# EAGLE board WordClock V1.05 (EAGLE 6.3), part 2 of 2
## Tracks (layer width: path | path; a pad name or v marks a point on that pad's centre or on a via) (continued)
LED13@U1  (via drill 0.5) (continued)
  Bottom 0.254: U101.27 145.25,352.19 145.77,351.66 v145.77,350.65
LED13@U2  (via drill 0.5)
  Top 0.406: v145.77,288.65 146.03,288.39 234.29,288.39 238.86,283.82 238.86,283.33 D220.C
  Bottom 0.254: U201.27 145.25,290.19 145.77,289.66 v145.77,288.65
LED13@U3  (via drill 0.5)
  Top 0.406: v145.77,226.65 146.03,226.39 234.29,226.39 238.86,221.82 238.86,221.33 D320.C
  Bottom 0.254: U301.27 145.25,228.19 145.77,227.66 v145.77,226.65
LED13@U4  (via drill 0.5)
  Top 0.406: v145.77,164.65 146.03,164.39 234.29,164.39 238.86,159.82 238.86,159.33 D420.C
  Bottom 0.254: U401.27 145.25,166.19 145.77,165.66 v145.77,164.65
LED13@U5  (via drill 0.5)
  Top 0.406: v145.77,102.65 146.03,102.39 154.44,102.39 156.44,104.39 156.44,110.49 158.34,112.39 237.59,112.39 239.3,110.69 D520.C
  Bottom 0.254: U501.27 145.25,104.19 145.77,103.66 v145.77,102.65
LED14@U1  (via drill 0.5)
  Top 0.406: v145.01,351.41 145.01,350.14 145.52,349.63 207.11,349.63 211.18,345.57 211.18,344.91 D119.C
  Bottom 0.254: U101.28 144.75,351.67 v145.01,351.41
LED14@U2  (via drill 0.5)
  Top 0.406: v145.01,289.41 145.01,288.14 145.52,287.63 207.11,287.63 211.18,283.57 211.18,282.91 D219.C
  Bottom 0.254: U201.28 144.75,289.67 v145.01,289.41
LED14@U3  (via drill 0.5)
  Top 0.406: v145.01,227.41 145.01,226.14 145.52,225.63 207.11,225.63 211.18,221.57 211.18,220.91 D319.C
  Bottom 0.254: U301.28 144.75,227.67 v145.01,227.41
LED14@U4  (via drill 0.5)
  Top 0.406: v145.01,165.41 145.01,164.14 145.52,163.63 207.11,163.63 211.18,159.57 211.18,158.91 D419.C
  Bottom 0.254: U401.28 144.75,165.67 v145.01,165.41
LED14@U5  (via drill 0.5)
  Top 0.406: v145.01,103.41 145.01,102.14 145.52,101.63 207.11,101.63 211.18,97.57 211.18,96.91 D519.C
  Bottom 0.254: U501.28 144.75,103.67 v145.01,103.41
LED15@U1  (via drill 0.5)
  Top 0.406: D118.C 182.86,345.13 182.86,345.69 179.81,348.74 145.26,348.74 144.25,349.76 v144.25,350.64 v144.25,350.65
  Bottom 0.254: U101.29 v144.25,350.65
LED15@U2  (via drill 0.5)
  Top 0.406: D218.C 182.86,283.13 182.86,283.69 179.81,286.74 145.26,286.74 144.25,287.76 144.25,288.01 144.25,288.02 v144.25,288.65
  Bottom 0.254: U201.29 v144.25,288.65
LED15@U3  (via drill 0.5)
  Top 0.406: D318.C 182.86,221.13 182.86,221.69 179.81,224.74 145.26,224.74 144.25,225.76 v144.25,226.64 v144.25,226.65
  Bottom 0.254: U301.29 v144.25,226.65
LED15@U4  (via drill 0.5)
  Top 0.406: v144.25,164.65 144.25,163.76 145.26,162.74 179.81,162.74 182.86,159.69 182.86,159.13 D418.C
  Bottom 0.254: U401.29 v144.25,164.65
LED15@U5  (via drill 0.5)
  Top 0.406: D518.C 182.86,97.13 182.86,97.69 179.81,100.74 145.26,100.74 144.25,101.76 v144.25,102.64 v144.25,102.65
  Bottom 0.254: U501.29 v144.25,102.65
LED16@U1  (via drill 0.5)
  Top 0.406: D117.C 154.92,344.97 154.92,345.57 152.5,347.98 144.76,347.98 142.75,349.99 142.75,351.38 v142.72,351.41
  Bottom 0.254: U101.32 142.75,351.44 v142.72,351.41
LED16@U2  (via drill 0.5)
  Top 0.406: v142.75,289.41 142.75,287.99 144.76,285.98 152.5,285.98 154.92,283.57 154.92,282.97 D217.C
  Bottom 0.254: U201.32 v142.75,289.41 142.72,289.41
LED16@U3  (via drill 0.5)
  Top 0.406: D317.C 154.92,220.97 154.92,221.57 152.5,223.98 144.76,223.98 142.75,225.99 142.75,227.38 v142.72,227.41
  Bottom 0.254: U301.32 142.75,227.44 v142.72,227.41
LED16@U4  (via drill 0.5)
  Top 0.406: v142.75,165.41 142.75,163.99 144.76,161.98 152.5,161.98 154.92,159.57 154.92,158.97 D417.C
  Bottom 0.254: U401.32 v142.75,165.41 142.72,165.41
LED16@U5  (via drill 0.5)
  Top 0.406: D517.C 154.92,96.97 154.92,97.57 152.5,99.98 144.76,99.98 142.75,101.99 142.75,103.38 v142.72,103.41
  Bottom 0.254: U501.32 142.75,103.44 v142.72,103.41
LED17@U1  (via drill 0.5)
  Top 0.406: 126.9,344.28 D116.C 127.48,345.47 127.48,346.2 130.15,348.87 141.07,348.87 141.96,349.76 v141.96,350.65
  Bottom 0.254: U101.33 142.25,351.95 141.96,351.66 v141.96,350.65
LED17@U2  (via drill 0.5)
  Top 0.406: 126.9,282.28 D216.C 127.48,283.47 127.48,284.2 130.15,286.87 141.07,286.87 141.96,287.76 v141.96,288.65
  Bottom 0.254: U201.33 142.25,289.95 141.96,289.66 v141.96,288.65
LED17@U3  (via drill 0.5)
  Top 0.406: 126.9,220.28 D316.C 127.48,221.47 127.48,222.2 130.15,224.87 141.07,224.87 141.96,225.76 v141.96,226.65
  Bottom 0.254: U301.33 142.25,227.95 141.96,227.66 v141.96,226.65
LED17@U4  (via drill 0.5)
  Top 0.406: 126.9,158.28 D416.C 127.48,159.47 127.48,160.2 130.15,162.87 141.07,162.87 141.96,163.76 v141.96,164.65
  Bottom 0.254: U401.33 142.25,165.95 141.96,165.66 v141.96,164.65
LED17@U5  (via drill 0.5)
  Top 0.406: 126.9,96.28 D516.C 127.48,97.47 127.48,98.2 130.15,100.87 141.07,100.87 141.96,101.76 v141.96,102.65
  Bottom 0.254: U501.33 142.25,103.95 141.96,103.66 v141.96,102.65
LED18@U1  (via drill 0.5)
  Top 0.406: v141.2,351.41 141.2,350.14 140.82,349.76 102.72,349.76 98.78,345.82 98.78,344.91 D115.C
  Bottom 0.254: U101.34 141.75,352.21 141.2,351.66 v141.2,351.41
LED18@U2  (via drill 0.5)
  Top 0.406: v141.2,289.41 141.2,288.14 140.82,287.76 102.72,287.76 98.78,283.82 98.78,282.91 D215.C
  Bottom 0.254: U201.34 141.75,290.21 141.2,289.66 v141.2,289.41
LED18@U3  (via drill 0.5)
  Top 0.406: v141.2,227.41 141.2,226.14 140.82,225.76 102.72,225.76 98.78,221.82 98.78,220.91 D315.C
  Bottom 0.254: U301.34 141.75,228.21 141.2,227.66 v141.2,227.41
LED18@U4  (via drill 0.5)
  Top 0.406: v141.2,165.41 141.2,164.14 140.82,163.76 102.72,163.76 98.78,159.82 98.78,158.91 D415.C
  Bottom 0.254: U401.34 141.75,166.21 141.2,165.66 v141.2,165.41
LED18@U5  (via drill 0.5)
  Top 0.406: v141.2,103.41 141.2,102.14 140.82,101.76 102.72,101.76 98.78,97.82 98.78,96.91 D515.C
  Bottom 0.254: U501.34 141.75,104.21 141.2,103.66 v141.2,103.41
LED19@U1  (via drill 0.5)
  Top 0.406: v140.44,350.65 75.54,350.65 70.84,345.95 70.84,345.03 D114.C
  Bottom 0.254: U101.35 141.25,352.48 140.44,351.66 v140.44,350.65
LED19@U2  (via drill 0.5)
  Top 0.406: v140.44,288.65 75.54,288.65 70.84,283.95 70.84,283.03 D214.C
  Bottom 0.254: U201.35 141.25,290.48 140.44,289.66 v140.44,288.65
LED19@U3  (via drill 0.5)
  Top 0.406: v140.44,226.65 75.54,226.65 70.84,221.95 70.84,221.03 D314.C
  Bottom 0.254: U301.35 141.25,228.48 140.44,227.66 v140.44,226.65
LED19@U4  (via drill 0.5)
  Top 0.406: v140.44,164.65 75.54,164.65 70.84,159.95 70.84,159.03 D414.C
  Bottom 0.254: U401.35 141.25,166.47 140.44,165.66 v140.44,164.65
LED19@U5  (via drill 0.5)
  Top 0.406: v140.44,102.65 75.54,102.65 70.84,97.95 70.84,97.03 D514.C
  Bottom 0.254: U501.35 141.25,104.47 140.44,103.66 v140.44,102.65
LED20@U1  (via drill 0.5)
  Top 0.406: v137.14,357 53.7,357 42.77,346.07 42.77,345.06 D113.C
  Bottom 0.254: U101.41 v137.14,356.99 v137.14,357
LED20@U2  (via drill 0.5)
  Top 0.406: v137.14,295 53.7,295 42.77,284.07 42.77,283.06 D213.C
  Bottom 0.254: U201.41 v137.14,294.99 v137.14,295
LED20@U3  (via drill 0.5)
  Top 0.406: v137.14,233 53.7,233 42.77,222.07 42.77,221.06 D313.C
  Bottom 0.254: U301.41 v137.14,232.99 v137.14,233
LED20@U4  (via drill 0.5)
  Top 0.406: v137.14,171 53.7,171 42.77,160.07 42.77,159.06 D413.C
  Bottom 0.254: U401.41 v137.14,170.99 v137.14,171
LED20@U5  (via drill 0.5)
  Top 0.406: v137.14,109 53.7,109 42.77,98.07 42.77,97.06 D513.C
  Bottom 0.254: U501.41 v137.14,108.99 v137.14,109
LED21@U1  (via drill 0.5)
  Top 0.406: D112.C 14.56,344.95 14.56,353.04 23.98,362.46 131.8,362.46 v136.5,357.76
  Bottom 0.254: U101.42 137.79,357.49 137.52,357.76 v136.5,357.76
LED21@U2  (via drill 0.5)
  Top 0.406: v136.5,295.76 26.38,295.76 14.56,283.95 14.56,282.95 D212.C
  Bottom 0.254: U201.42 137.79,295.49 137.52,295.76 v136.5,295.76
LED21@U3  (via drill 0.5)
  Top 0.406: v136.5,233.76 131.79,238.46 23.94,238.46 14.5,229.03 D312.C 14.56,220.95
  Bottom 0.254: U301.42 137.79,233.49 137.52,233.76 v136.5,233.76
LED21@U4  (via drill 0.5)
  Top 0.406: v136.5,171.76 26.38,171.76 14.56,159.95 14.56,158.95 D412.C
  Bottom 0.254: U401.42 137.79,171.49 137.52,171.76 v136.5,171.76
LED21@U5  (via drill 0.5)
  Top 0.406: v136.5,109.76 v136.5,109.75 131.87,114.38 24.21,114.38 14.56,104.73 14.56,96.95 D512.C
  Bottom 0.254: U501.42 137.79,109.49 137.52,109.76 v136.5,109.76
MATRIX-OE#  (via drill 0.5)
  Top 0.254: v159.62,104.14 225.4,104.14 v225.78,103.76
  Bottom 0.254: U101.24 148.92,354.99 151.61,352.3 151.61,292.99 | 151.61,230.99 151.61,292.99 | 151.61,230.99 151.61,169.01 | U401.24 151.59,168.99 151.61,169.01 | U301.24 151.61,230.99 | U201.24 151.61,292.99 | 151.61,169.01 151.61,107.01 | 151.61,107.01 151.61,106.43 153.9,104.14 v159.62,104.14 | U501.24 151.59,106.99 151.61,107.01 | U704.55 225.72,103.7 v225.78,103.76
MATRIX-PWR  (via drill 0.5)
  Top 0.254: v276.07,68.58 U601.3 | v254.74,78.1 v276.07,78.1
  Bottom 0.254: v276.07,78.1 v276.07,68.58 | v254.74,78.1 253.98,78.87 253.98,88.38 248.77,93.58 U704.9
MATRIX-SCL  (via drill 0.5)
  Top 0.254: v233.17,79.25 232.79,79.63 158.6,79.63 v158.34,79.38
  Bottom 0.254: R113.1 158.98,353.06 160.63,351.41 160.63,291.08 | 160.63,229.36 160.63,291.08 | 160.63,229.36 160.63,167.39 | 160.63,167.39 160.63,105.41 | 160.63,291.08 R213.1 | R313.1 160.63,229.36 | 160.63,167.39 R413.1 | 160.63,105.41 R513.1 | v233.17,79.25 R710.1 | 160.63,105.41 160.63,83.82 160.15,83.34 R706.2 158.34,79.44 v158.34,79.38
MATRIX-SDA  (via drill 0.5)
  Top 0.254: v161.77,293.12 v159.74,293.12 | v159.79,231.37 v161.77,231.37 | v161.77,169.42 v159.87,169.42 | v161.77,107.44 v158.85,107.44 | v235.21,79.25 234.29,79.25 233.6,78.56 232.69,78.56 232.06,79.2 164.75,79.2 v164.44,78.89
  Bottom 0.254: R112.1 158.37,355.07 161.9,351.54 v161.77,293.12 v161.77,231.37 v161.77,169.42 v161.77,107.44 161.77,83.82 162.18,83.41 R707.2 162.19,81.23 163.73,81.23 164.44,80.52 v164.44,78.89 | v159.74,293.12 R212.1 | R312.1 v159.79,231.37 | v159.87,169.42 R412.1 | v235.21,79.25 R709.1 | v158.85,107.44 R512.1
N$1
  Bottom 0.254: U704.16 234.47,87.98 234.47,86.36 235.21,85.62 R709.2
N$2
  Bottom 0.254: U704.17 232.93,82.38 R710.2
N$3
  Top 0.406: U603.3 246.86,66.04 247.88,65.02 250.67,65.02 251.4,64.3 R611.1 252.2,64.01 252.58,63.63 252.58,60.32 252.2,59.94 R608.2
N$4
  Top 0.406: U603.6 249.44,69.85 R610.2 | R610.2 C605.2 | R610.2 R609.2 R612.1
N$5
  Top 0.406: R603.2 274.73,58.73 274.17,58.17 271.5,58.17 | R603.3 271.5,57.73 271.5,58.17 | U601.6 275.82,64.77 275.06,65.53 271.16,65.53 | C601.2 271.12,64.55 | C601.2 271.16,65.53 | 271.16,65.53 R604.1 | 271.5,58.17 269.85,58.17 269.34,58.67 269.34,64.01 269.85,64.52 C601.2
N$6
  Top 0.406: U601.5 276.07,66.04 273.53,68.58 C603.1
N$7
  Top 0.406: U601.2 272.43,69.85 R601.2
N$8
  Top 0.406: C612.1 248.51,66.04 245.97,68.58 U603.5
N$9  (via drill 0.5)
  Top 0.254: v236.32,105.28 231.07,105.28 226.53,100.73 v226.53,99.52
  Bottom 0.254: J703.1 257.66,76.71 257.66,97.48 249.86,105.28 v236.32,105.28 | v226.53,99.52 U704.56
N$10
  Top 0.406: R607.2 251.4,62.27 250.67,62.99 247.88,62.99 246.1,64.77 U603.2
N$11  (via drill 0.5, 0.6)
  Top 0.254: v235.56,104.52 231.39,104.52 227.32,100.53 v227.32,100.28 | v251.06,80.64 v256.77,80.64
  Bottom 0.254: v235.56,104.52 249.57,104.52 256.9,97.19 256.9,80.64 | 256.9,80.64 J703.5 | U703.1 213.02,106.89 214.61,108.48 214.8,108.48 R704.2 219.16,104.75 226.06,104.75 226.87,103.94 226.87,102.72 227.32,102.27 U704.57 v227.32,100.28 | J704.6 249.78,81.28 250.42,80.64 v251.06,80.64 | v256.77,80.64 256.9,80.64
N$12
  Bottom 0.254: C707.1 230.34,106.45 XTAL701.3 228.3,106.32 228.3,102.89 228.93,102.27 U704.59
N$13
  Bottom 0.254: C706.1 220.21,108.95 XTAL701.1 222.25,108.95 222.84,108.36 225,108.36 226.67,106.68 226.67,105.28 227.56,104.39 227.56,102.87 228.12,102.3 U704.58
N$14  (via drill 0.5)
  Top 0.254: U602.17 170.41,68.42 170.64,68.2 170.64,67.28 v170.54,67.16
  Bottom 0.254: v170.54,67.16 170.46,67.23 170.46,68.87 C610.1
N$15  (via drill 0.5)
  Top 0.406: L601.2 v168.25,71.12 168.46,70.91 U602.20
  Bottom 0.254: C608.1 166.92,67.85 165.58,66.52 165.58,66.36 R606.1
  Bottom 0.406: 167.24,71.12 166.86,71.12 C607.1 | 167.24,71.12 v168.25,71.12 | C608.1 166.92,70.8 167.24,71.12
N$16
  Top 0.406: XTAL801.2 39.22,61.72 U801.5
N$19
  Top 0.406: X503.1 D523.C
N$20
  Top 0.406: XTAL801.1 38.71,60.45 U801.6
N$21
  Top 0.406: U801.13 53.19,62.99 XTAL802.2
N$22
  Top 0.406: U801.14 52.94,64.26 XTAL802.1
N$23
  Top 0.254: C805.1 38.16,66.8
  Top 0.406: 38.16,66.8 U801.1 42.01,66.8 42.39,67.18 | C805.1 C804.1 33.67,66.89 X801.1 | 42.39,67.18 C806.1 44.14,69.46 C807.1 44.78,70.1 44.93,70.1 45.99,71.16 R802.1 | U801.12 47.85,61.72 42.39,67.18
N$24
  Top 0.406: R802.2 48.23,69.46 C808.1 52.8,69.72 J801.4 52.94,73.02 53.57,73.66 59.32,73.66 R801.1
N$25
  Top 0.406: U801.7 38.81,59.18 38.41,58.78 38.09,58.78 C801.1
N$26
  Top 0.406: C802.1 54.29,56.77 49,56.77 47.85,57.91 U801.8 C801.2
N$27
  Top 0.406: U801.9 C802.2
N$28
  Top 0.406: U801.10 54.17,59.18 C803.1
N$29
  Top 0.406: U801.11 C803.2
N$30  (via drill 0.5)
  Top 0.406: v49,65.53 U801.15
  Bottom 0.406: J801.3 54.2,68.83 53.44,68.07 49.25,68.07 48.62,67.44 48.62,65.91 v49,65.53
N$31
  Top 0.406: U801.2 38.42,65.53 C805.2 C804.2 32.02,65.19 X802.1
N$32
  Top 0.406: J801.2 56.49,68.83 61.32,68.83 Q801.3 61.32,69.57 61.75,70 61.75,72.1 R801.2
N$33
  Top 0.406: R803.2 59.94,66.8 Q801.1
N$34
  Top 0.406: U801.16 R803.1
N$36
  Bottom 0.406: R701.2 194.96,157.39 194.84,157.28 | 194.84,157.28 C701.1 | 194.84,157.28 193.22,157.28 U701.1
N$38  (via drill 0.5)
  Top 0.406: v136.88,133.98 137.77,134.87 138.41,134.87 138.53,134.75 309.48,134.75 312.01,132.21 312.01,81.28 J501.2 309.86,77.09 309.86,71.25 J501A.2
  Bottom 0.254: U501.43 138.02,109.99 137.21,110.79
  Bottom 0.406: 137.21,110.79 137.21,133.15 136.88,133.48 v136.88,133.98
N$39
  Bottom 0.61: R703.2 303.9,114.56 C703.1 U702.2
N$40  (via drill 0.5)
  Top 0.406: v150.61,69.04 D523.A
  Bottom 0.406: R525.2 150.61,62.08 v150.61,69.04
N$41  (via drill 0.5)
  Top 0.406: v138.03,133.98 309.09,133.98 311.13,131.95 311.13,82.93 J501.4
  Bottom 0.254: U501.44 138.41,110.49 138.03,110.87
  Bottom 0.406: v138.03,133.98 138.03,110.87 | J501.4 310.11,79.38 310.11,68.96 J501A.4
N$42
  Bottom 0.406: R525.1 150.61,60.38 X501.1
N$44
  Bottom 0.406: R526.1 X502.1
N$45  (via drill 0.5)
  Top 0.406: v134.61,62.04 v134.6,62.04 D524.C
  Bottom 0.406: v134.61,62.04 X504.1
N$46  (via drill 0.5)
  Top 0.406: v130.61,62.14 v130.6,62.14 D524.A
  Bottom 0.406: v130.61,62.14 R526.2
N$47
  pour Top: 138.91,75.24 138.91,55.84 156.91,55.84 156.91,75.24
  pour Top: 118.91,75.24 118.91,55.84 136.91,55.84 136.91,75.24
  pour Top: 98.91,75.24 98.91,55.84 116.91,55.84 116.91,75.24
  pour Top: 78.91,75.24 78.91,55.84 96.91,55.84 96.91,75.24
  pour Bottom: 78.91,75.24 78.91,55.84 96.91,55.84 96.91,75.24
  pour Bottom: 98.91,75.24 98.91,55.84 116.91,55.84 116.91,75.24
  pour Bottom: 118.91,75.24 118.91,55.84 136.91,55.84 136.91,75.24
  pour Bottom: 138.91,75.24 138.91,55.84 156.91,55.84 156.91,75.24
N$48  (via drill 0.5)
  Top 0.406: v137.14,172.59 16.61,172.59 6.58,162.56 6.58,83.44 8.87,81.15 8.87,79.12 J401.2 8.87,77.09 8.87,70.61 J401A.2
  Bottom 0.254: U401.43 138.12,171.99 137.52,172.59 v137.14,172.59
N$49
  Bottom 0.406: U901.27 245.34,29.5 C903.2
N$50
  Bottom 0.406: U901.28 242.8,29.5 C903.1
N$51
  Bottom 0.406: U901.29 240.26,29.5 C902.2
N$52
  Bottom 0.406: U901.30 237.72,29.5 C902.1
N$53
  Bottom 0.406: C901.1 U901.32 U901.31
N$54  (via drill 0.5)
  Top 0.406: v136.5,173.48 15.98,173.35 5.56,162.94 5.56,82.93 J401.4 4.8,80.64 4.04,79.88 4.04,67.69 4.67,67.06 J401A.4
  Bottom 0.254: U401.44 138.51,172.49 137.52,173.48 v136.5,173.48
N$55
  Top 0.406: X403.1 D423.C
N$56  (via drill 0.5)
  Top 0.406: v101.31,69.04 D423.A
  Bottom 0.406: R425.2 v101.31,69.04
N$57
  Bottom 0.406: X401.1 R425.1
N$58
  Bottom 0.406: R426.1 X402.1
N$60  (via drill 0.5)
  Top 0.406: D424.C v85.21,62.04
  Bottom 0.406: v85.21,62.04 X404.1
N$62  (via drill 0.5)
  Top 0.406: v81.21,62.04 D424.A
  Bottom 0.406: v81.21,62.04 R426.2
N$69
  Top 1.016: J603.2 188.06,69.85 | 188.06,69.85 J603.1 189.84,71.63 196.22,71.63 J601.1 | 188.06,69.85 J603.3
N$70  (via drill 0.5)
  Top 0.254: v163.93,58.67 163.26,59.34 U602.1
  Bottom 0.254: J603.5 184.25,59.94 182.98,58.67 v163.93,58.67
N$71  (via drill 0.5)
  Top 0.254: v166.47,59.44 165.86,60.04 U602.5
  Bottom 0.254: J603.7 181.71,66.04 183.49,64.26 183.49,60.2 182.73,59.44 v166.47,59.44
N$73
  Top 0.406: R602.2 271.16,60.47 R603.1
N$87  (via drill 0.5)
  Top 0.406: L601.1 173.2,71.12 | 173.2,71.12 C606.1 | 173.2,71.12 v173.2,69.98 | J602.1 177.57,62.28 178.16,61.7 v178.54,61.7
  Bottom 0.406: v173.2,69.98 178.16,69.98 179.17,68.96 179.17,67.82 179.94,67.06 179.94,62.08 179.55,61.7 v178.54,61.7
N$88  (via drill 0.5)
  Top 0.254: U602.19 169.11,68.3 168.76,67.94 v168.76,67.16
  Bottom 0.254: v168.76,67.16 168.76,66.08 R605.2 R606.2
PA3
  Bottom 0.254: U704.1 243.72,99.98 245.97,102.23 X9.P$1
PA4
  Bottom 0.254: U704.2 244.19,99.18 245.97,100.97 X10.P$1
PA5
  Bottom 0.254: U704.3 244.66,98.38 245.97,99.69 X11.P$1
PA6
  Bottom 0.254: U704.4 245.76,97.58 246.61,98.42 X12.P$1
PA7
  Bottom 0.254: U704.5 246.87,96.78 X13.P$1
PB0
  Bottom 0.254: U704.6 248.61,95.98 X14.P$1
PB4  (via drill 0.6)
  Top 0.254: X15.P$1 249.15,92.07 249.78,91.44 v249.78,89.53
  Bottom 0.254: U704.10 245.91,92.78 X15.P$1 | v249.78,89.53 J704.5
PB5
  Bottom 0.254: U704.11 235.21,91.98 235.43,92.2 243.82,92.2 245.21,90.8 X16.P$1 249.78,90.8 252.32,88.27 J704.9
PB6  (via drill 0.6)
  Top 0.254: X17.P$1 246.61,88.27 v245.34,86.99
  Bottom 0.254: U704.12 235.22,91.18 235.61,91.57 243.31,91.57 245.34,89.53 X17.P$1 | v245.34,86.99 245.34,86.36 245.78,85.92 J704.1
PB7
  Bottom 0.254: U704.13 235.21,90.38 235.84,91.01 242.85,91.01 245.59,88.27 X18.P$1 J704.3
PE0
  Bottom 0.254: U704.36 218.64,90.38 218.03,90.98 206.66,90.98 204.57,88.9 X1.P$1
PE1
  Bottom 0.254: X2.P$1 204.7,90.17 206.13,91.6 218.2,91.6 218.62,91.18 U704.37
PE2
  Bottom 0.254: U704.38 218.69,91.98 218.52,92.15 204.78,92.15 X3.P$1
PE3
  Bottom 0.254: U704.39 201.59,92.78 X4.P$1
PE4
  Bottom 0.254: U704.40 204.47,93.58 X5.P$1
PE5
  Bottom 0.254: X6.P$1 204.45,95.25 205.53,94.17 218.43,94.17 218.64,94.38 U704.41
PE6
  Bottom 0.254: U704.42 218.62,95.18 218.21,94.77 206.07,94.77 204.32,96.52 X7.P$1
PE7
  Bottom 0.254: U704.43 218.64,95.98 218.06,95.4 206.83,95.4 204.45,97.79 X8.P$1
PIR  (via drill 0.5)
  Top 0.254: v195.68,111.48 v231.9,111.48
  Bottom 0.254: v195.68,111.48 195.68,144.65 189.71,150.62 U701.2 | U704.62 231.32,102.29 231.9,102.87 v231.9,111.48
  Bottom 0.406: C702.1 U701.2 R702.1 191.28,155.79 190.98,156.08
R1@U1
  Top 0.406: R101.2 15.65,377.04 D101.A
R1@U2
  Top 0.406: R201.2 15.65,315.04 D201.A
R1@U3
  Top 0.406: R301.2 15.65,253.04 D301.A
R1@U4
  Top 0.406: R401.2 15.65,191.04 D401.A
R1@U5
  Top 0.406: R501.2 15.65,129.04 D501.A
R2@U1
  Top 0.406: R102.2 43.75,377.04 D102.A
R2@U2
  Top 0.406: R202.2 43.75,315.04 D202.A
R2@U3
  Top 0.406: R302.2 43.75,253.04 D302.A
R2@U4
  Top 0.406: R402.2 43.75,191.04 D402.A
R2@U5
  Top 0.406: R502.2 43.75,129.04 D502.A
R3@U1
  Top 0.406: R103.2 71.85,377.04 D103.A
R3@U2
  Top 0.406: R203.2 71.85,315.04 D203.A
R3@U3
  Top 0.406: R303.2 71.85,253.04 D303.A
R3@U4
  Top 0.406: R403.2 71.85,191.04 D403.A
R3@U5
  Top 0.406: R503.2 71.85,129.04 D503.A
R4@U1
  Top 0.406: R104.2 99.95,377.04 D104.A
R4@U2
  Top 0.406: R204.2 99.95,315.04 D204.A
R4@U3
  Top 0.406: R304.2 99.95,253.04 D304.A
R4@U4
  Top 0.406: R404.2 99.95,191.04 D404.A
R4@U5
  Top 0.406: R504.2 99.95,129.04 D504.A
R5@U1
  Top 0.406: R105.2 128.05,377.04 D105.A
R5@U2
  Top 0.406: R205.2 128.05,315.04 D205.A
R5@U3
  Top 0.406: R305.2 128.05,253.04 D305.A
R5@U4
  Top 0.406: R405.2 128.05,191.04 D405.A
R5@U5
  Top 0.406: R505.2 128.05,129.04 D505.A
R6@U1
  Top 0.406: R106.2 156.15,377.04 D106.A
R6@U2
  Top 0.406: R206.2 156.15,315.04 D206.A
R6@U3
  Top 0.406: R306.2 156.15,253.04 D306.A
R6@U4
  Top 0.406: R406.2 156.15,191.04 D406.A
R6@U5
  Top 0.406: R506.2 156.15,129.04 D506.A
R7@U1
  Top 0.406: R107.2 184.25,377.04 D107.A
R7@U2
  Top 0.406: R207.2 184.25,315.04 D207.A
R7@U3
  Top 0.406: R307.2 184.25,253.04 D307.A
R7@U4
  Top 0.406: R407.2 184.25,191.04 D407.A
R7@U5
  Top 0.406: R507.2 184.25,129.04 D507.A
R8@U1
  Top 0.406: R108.2 212.35,377.04 D108.A
R8@U2
  Top 0.406: R208.2 212.35,315.04 D208.A
R8@U3
  Top 0.406: R308.2 212.35,253.04 D308.A
R8@U4
  Top 0.406: R408.2 212.35,191.04 D408.A
R8@U5
  Top 0.406: R508.2 212.35,129.04 D508.A
R9@U1
  Top 0.406: R109.2 240.45,377.04 D109.A
R9@U2
  Top 0.406: R209.2 240.45,315.04 D209.A
R9@U3
  Top 0.406: R309.2 240.45,253.04 D309.A
R9@U4
  Top 0.406: R409.2 240.45,191.04 D409.A
R9@U5
  Top 0.406: R509.2 240.45,129.04 D509.A
R10@U1
  Top 0.406: R110.2 268.55,377.04 D110.A
R10@U2
  Top 0.406: R210.2 268.55,315.04 D210.A
R10@U3
  Top 0.406: R310.2 268.55,253.04 D310.A
R10@U4
  Top 0.406: R410.2 268.55,191.04 D410.A
R10@U5
  Top 0.406: R510.2 268.55,129.04 D510.A
R11@U1
  Top 0.406: R111.2 296.65,377.04 D111.A
R11@U2
  Top 0.406: R211.2 296.65,315.04 D211.A
R11@U3
  Top 0.406: R311.2 296.65,253.04 D311.A
R11@U4
  Top 0.406: R411.2 296.65,191.04 D411.A
R11@U5
  Top 0.406: R511.2 296.65,129.04 D511.A
R12@U1
  Top 0.406: R114.1 17.35,337.44 D112.A
R12@U2
  Top 0.406: R214.1 17.35,275.44 D212.A
R12@U3
  Top 0.406: R314.1 17.35,213.44 D312.A
R12@U4
  Top 0.406: R414.1 17.35,151.44 D412.A
R12@U5
  Top 0.406: R514.1 17.35,89.44 D512.A
R13@U1
  Top 0.406: R115.1 45.45,337.44 D113.A
R13@U2
  Top 0.406: R215.1 45.45,275.44 D213.A
R13@U3
  Top 0.406: R315.1 45.45,213.44 D313.A
R13@U4
  Top 0.406: R415.1 45.45,151.44 D413.A
R13@U5
  Top 0.406: R515.1 45.45,89.44 D513.A
R14@U1
  Top 0.406: R116.1 73.55,337.44 D114.A
R14@U2
  Top 0.406: R216.1 73.55,275.44 D214.A
R14@U3
  Top 0.406: R316.1 73.55,213.44 D314.A
R14@U4
  Top 0.406: R416.1 73.55,151.44 D414.A
R14@U5
  Top 0.406: R516.1 73.55,89.44 D514.A
R15@U1
  Top 0.406: R117.1 101.65,337.44 D115.A
R15@U2
  Top 0.406: R217.1 101.65,275.44 D215.A
R15@U3
  Top 0.406: R317.1 101.65,213.44 D315.A
R15@U4
  Top 0.406: R417.1 101.65,151.44 D415.A
R15@U5
  Top 0.406: R517.1 101.65,89.44 D515.A
R16@U1
  Top 0.406: R118.1 129.75,338.59 D116.A
R16@U2
  Top 0.406: R218.1 129.75,276.59 D216.A
R16@U3
  Top 0.406: R318.1 129.75,214.59 D316.A
R16@U4
  Top 0.406: R418.1 129.75,152.59 D416.A
R16@U5
  Top 0.406: R518.1 129.75,90.59 D516.A
R17@U1
  Top 0.406: R119.1 157.85,338.59 D117.A
R17@U2
  Top 0.406: R219.1 157.85,276.59 D217.A
R17@U3
  Top 0.406: R319.1 157.85,214.59 D317.A
R17@U4
  Top 0.406: R419.1 157.85,152.59 D417.A
R17@U5
  Top 0.406: R519.1 157.85,90.59 D517.A
R18@U1
  Top 0.406: R120.1 185.95,338.59 D118.A
R18@U2
  Top 0.406: R220.1 185.95,276.59 D218.A
R18@U3
  Top 0.406: R320.1 185.95,214.59 D318.A
R18@U4
  Top 0.406: R420.1 185.95,152.59 D418.A
R18@U5
  Top 0.406: R520.1 185.95,90.59 D518.A
R19@U1
  Top 0.406: R121.1 214.05,338.59 D119.A
R19@U2
  Top 0.406: R221.1 214.05,276.59 D219.A
R19@U3
  Top 0.406: R321.1 214.05,214.59 D319.A
R19@U4
  Top 0.406: R421.1 214.05,152.59 D419.A
R19@U5
  Top 0.406: R521.1 214.05,90.59 D519.A
R20@U1
  Top 0.406: R122.1 242.15,338.59 D120.A
R20@U2
  Top 0.406: R222.1 242.15,276.59 D220.A
R20@U3
  Top 0.406: R322.1 242.15,214.59 D320.A
R20@U4
  Top 0.406: R422.1 242.15,152.59 D420.A
R20@U5
  Top 0.406: R522.1 242.15,90.59 D520.A
R21@U1
  Top 0.406: R123.1 270.25,338.59 D121.A
R21@U2
  Top 0.406: R223.1 270.25,276.59 D221.A
R21@U3
  Top 0.406: R323.1 270.25,214.59 D321.A
R21@U4
  Top 0.406: R423.1 270.25,152.59 D421.A
R21@U5
  Top 0.406: R523.1 270.25,90.59 D521.A
R22@U1
  Top 0.406: R124.1 298.35,338.59 D122.A
R22@U2
  Top 0.406: R224.1 298.35,276.59 D222.A
R22@U3
  Top 0.406: R324.1 298.35,214.59 D322.A
R22@U4
  Top 0.406: R424.1 298.35,152.59 D422.A
R22@U5
  Top 0.406: R524.1 298.35,90.59 D522.A
RCV-EN#  (via drill 0.5, 0.6)
  Top 0.254: v254.74,79.63 v284.2,79.63 v296.14,79.63
  Bottom 0.254: v254.74,79.63 254.74,88.87 249.23,94.38 U704.8 | J701.3 226.93,385.83 227.81,386.72 309.09,386.72 310.62,385.19 310.62,142.24 308.08,139.7 291.06,139.7 289.15,137.79 289.15,107.31 284.2,102.36 v284.2,79.63 | v296.14,79.63 301.6,79.63 304.39,76.83 304.39,67.06 308.84,62.61 J701A.3
RESET#
  Top 0.406: U901.39 215.45,30.99 221.29,36.83 222.48,36.83 J901.4
RXD  (via drill 0.5)
  Top 0.254: v237.09,106.04 230.79,106.04 226.43,101.68 v220.01,101.68
  Bottom 0.254: J604.7 258.8,64.9 263.12,69.21 263.12,72.9 258.42,77.6 258.42,97.77 250.14,106.04 v237.09,106.04 | v220.01,101.68 220.82,101.68 U704.49
SCL@U1  (via drill 0.5)
  Top 0.254: v140.74,355.22 144.76,355.22 145.9,354.08 151.49,354.08 v151.74,353.82
  Bottom 0.254: U101.38 140.47,355.49 v140.74,355.22 | v151.74,353.82 152.5,353.06 R113.2
SCL@U2  (via drill 0.5)
  Top 0.254: v140.74,293.12 144.76,293.12 145.65,292.23 153.26,292.23 v154.41,291.08
  Bottom 0.254: U201.38 140.37,293.49 v140.74,293.12 | v154.41,291.08 R213.2
SCL@U3  (via drill 0.5)
  Top 0.254: v140.74,231.01 144.88,231.01 145.75,230.15 153.49,230.15 v154.28,229.36
  Bottom 0.254: U301.38 140.27,231.49 v140.74,231.01 | v154.28,229.36 R313.2
SCL@U4  (via drill 0.5)
  Top 0.254: v140.74,169.16 144.63,169.16 145.52,168.27 153.52,168.27 v154.41,167.39
  Bottom 0.254: U401.38 140.42,169.49 v140.74,169.16 | v154.41,167.39 R413.2
SCL@U5  (via drill 0.5)
  Top 0.254: v140.74,107.06 144.88,107.06 145.65,106.3 153.39,106.3 v154.28,105.41
  Bottom 0.254: U501.38 140.31,107.49 v140.74,107.06 | v154.28,105.41 R513.2
SDA@U1  (via drill 0.5)
  Top 0.254: v141.25,356.11 144.63,356.11 146.03,354.71 151.36,354.71 v151.72,355.07
  Bottom 0.254: U101.39 141.08,355.99 v141.25,356.11 | v151.72,355.07 R112.2
SDA@U2  (via drill 0.5)
  Top 0.254: v141.28,293.98 144.65,293.98 145.9,292.74 v154.41,292.74
  Bottom 0.254: U201.39 141.22,293.99 v141.28,293.98 | v154.41,292.74 154.79,293.12 R212.2
SDA@U3  (via drill 0.5)
  Top 0.254: v141.25,231.98 144.68,231.98 145.9,230.76 v154.26,230.76
  Bottom 0.254: U301.39 141.19,231.99 v141.25,231.98 | v154.26,230.76 154.87,231.37 R312.2
SDA@U4  (via drill 0.5)
  Top 0.254: v141.3,170 144.68,170 145.9,168.78 v154.41,168.78
  Bottom 0.254: U401.39 141.2,169.99 v141.3,170 | R412.2 155.55,169.42 155.17,169.04 154.66,169.04 v154.41,168.78
SDA@U5  (via drill 0.5)
  Top 0.254: v141.28,108 144.71,108 145.9,106.81 153.65,106.81 v154.28,107.44
  Bottom 0.254: U501.39 141.19,107.99 v141.28,108 | v154.28,107.44 R512.2
TL
  Top 0.406: S902.3 S902.4 207.03,25.4 207.03,29.25 212.32,34.54 215.11,34.54 J901.8
TR  (via drill 0.5)
  Top 0.406: 270.45,22.73 S904.3 | 270.45,22.73 S904.4 | v266.04,22.73 270.45,22.73
  Bottom 0.406: J901.10 216.13,36.83 211.05,31.75 211.05,29.21 217.52,22.73 v266.04,22.73
TXD  (via drill 0.5)
  Top 0.254: v237.85,106.81 230.64,106.81 226.07,102.23 220.45,102.23 220.32,102.36 219.69,102.36 219.08,101.76 v219.08,100.91
  Bottom 0.254: v237.85,106.81 250.37,106.81 259.18,97.99 259.18,77.85 263.75,73.28 263.75,68.96 261.34,66.55 J604.5 | v219.08,100.91 219.08,100.02 U704.48
V0
  Bottom 0.406: C906.1 U901.21
V1
  Bottom 0.406: C909.1 U901.22
V2
  Bottom 0.406: C907.1 U901.23
V3
  Bottom 0.406: C910.1 U901.24
V4
  Bottom 0.406: C908.1 U901.25
V+  (via drill 0.5)
  Top 0.406: U601.7 276.71,63.5 275.69,62.48 R602.1 C601.1
  Top 0.61: R111.1 298.35,380.19 297.54,381 270.11,381 | 242.29,381 270.11,381 | 214.1,381 242.29,381 | 186.03,381 214.1,381 | R110.1 270.25,380.86 270.11,381 | R109.1 242.15,380.86 242.29,381 | R108.1 214.05,380.95 214.1,381 | R107.1 185.95,380.92 186.03,381 | R101.1 18.61,381 45.57,381 | 73.64,381 45.57,381 | 101.7,381 73.64,381 | 129.77,381 101.7,381 | 157.96,381 163.42,381 C101.1 166.59,379.84 v166.6,379.86 v167.62,379.86 v168.63,379.86 | 157.96,381 129.77,381 | 186.03,381 178.62,381 C102.1 175.5,379.84 v175.49,379.86 v174.47,379.86 v173.46,379.86 | R105.1 129.75,380.98 129.77,381 | R104.1 101.65,380.95 101.7,381 | R103.1 73.55,380.91 73.64,381 | R102.1 45.45,380.88 45.57,381 | R114.2 17.02,333.38 43.79,333.38 | 71.86,333.38 43.79,333.38 | 100.18,333.38 71.86,333.38 | 128.12,333.38 100.18,333.38 | 156.19,333.38 164.01,333.38 C105.1 164.52,333.88 v166.6,333.88 v167.62,333.88 v168.63,333.88 | 156.19,333.38 128.12,333.38 | R118.2 128.05,333.37 128.12,333.38 | R117.2 99.95,333.38 100.18,333.38 | R115.2 43.75,333.42 43.79,333.38 | R116.2 71.85,333.38 71.86,333.38 | 268.58,333.25 295.16,333.25 R124.2 | 240.39,333.25 268.58,333.25 | 212.45,333.25 240.39,333.25 | 184.13,333.25 212.45,333.25 | 184.13,333.25 178.28,333.25 C106.1 177.64,333.88 v175.49,333.88 v174.47,333.88 v173.46,333.88 | R123.2 268.55,333.28 268.58,333.25 | R122.2 240.45,333.31 240.39,333.25 | R121.2 212.35,333.34 212.45,333.25 | R120.2 184.25,333.37 184.13,333.25 | R211.1 298.35,318.19 297.54,319 270.11,319 | 242.29,319 270.11,319 | 214.1,319 242.29,319 | 186.03,319 214.1,319 | R210.1 270.25,318.86 270.11,319 | R209.1 242.15,318.86 242.29,319 | R208.1 214.05,318.95 214.1,319
  Top 0.61: R207.1 185.95,318.92 186.03,319 | R201.1 18.61,319 45.57,319 | 73.64,319 45.57,319 | 101.7,319 73.64,319 | 129.77,319 101.7,319 | 157.84,319 129.77,319 | 157.84,319 163.42,319 C201.1 166.59,317.84 v166.6,317.86 v167.62,317.86 v168.63,317.86 | 186.03,319 178.62,319 C202.1 175.5,317.84 v175.49,317.86 v174.47,317.86 v173.46,317.86 | R205.1 129.75,318.98 129.77,319 | R204.1 101.65,318.95 101.7,319 | R203.1 73.55,318.91 73.64,319 | R202.1 45.45,318.88 45.57,319 | R214.2 17.02,271.38 43.79,271.38 | 71.86,271.38 43.79,271.38 | 100.18,271.38 71.86,271.38 | 128.12,271.38 100.18,271.38 | 156.19,271.38 128.12,271.38 | 156.19,271.38 164.01,271.38 C205.1 164.52,271.88 v166.6,271.88 v167.62,271.88 v168.63,271.88 | R218.2 128.05,271.37 128.12,271.38 | R217.2 99.95,271.38 100.18,271.38 | R215.2 43.75,271.42 43.79,271.38 | R216.2 71.85,271.38 71.86,271.38 | 268.58,271.25 295.16,271.25 R224.2 | 240.39,271.25 268.58,271.25 | 212.45,271.25 240.39,271.25 | 184.13,271.25 212.45,271.25 | 184.13,271.25 178.28,271.25 C206.1 177.64,271.88 v175.49,271.88 v174.47,271.88 v173.46,271.88 | R223.2 268.55,271.28 268.58,271.25 | R222.2 240.45,271.31 240.39,271.25 | R221.2 212.35,271.34 212.45,271.25 | R220.2 184.25,271.37 184.13,271.25 | R311.1 298.35,256.19 297.54,257 270.11,257 | 242.29,257 270.11,257 | 214.1,257 242.29,257 | 186.03,257 214.1,257 | R310.1 270.25,256.86 270.11,257 | R309.1 242.15,256.86 242.29,257 | R308.1 214.05,256.95 214.1,257 | R307.1 185.95,256.92 186.03,257 | R301.1 18.61,257 45.57,257 | 73.64,257 45.57,257 | 101.7,257 73.64,257 | 129.77,257 101.7,257 | 157.84,257 129.77,257 | 157.84,257 163.42,257 C301.1 166.59,255.84 v166.6,255.86 v167.62,255.86 v168.63,255.86
  Top 0.61: 186.03,257 178.49,257 C302.1 175.38,255.84 v175.36,255.86 v174.35,255.86 v173.33,255.86 | R305.1 129.75,256.98 129.77,257 | R304.1 101.65,256.95 101.7,257 | R303.1 73.55,256.91 73.64,257 | R302.1 45.45,256.88 45.57,257 | R314.2 17.02,209.38 43.79,209.38 | 71.86,209.38 43.79,209.38 | 100.18,209.38 71.86,209.38 | 128.12,209.38 100.18,209.38 | 156.06,209.38 128.12,209.38 | 156.06,209.38 164.01,209.38 C305.1 164.52,209.88 v166.6,209.88 v167.62,209.88 v168.63,209.88 | R318.2 128.05,209.37 128.12,209.38 | R317.2 99.95,209.38 100.18,209.38 | R315.2 43.75,209.42 43.79,209.38 | R316.2 71.85,209.38 71.86,209.38 | 268.58,209.25 295.16,209.25 R324.2 | 240.39,209.25 268.58,209.25 | 212.45,209.25 240.39,209.25 | 184.13,209.25 212.45,209.25 | 184.13,209.25 178.28,209.25 C306.1 177.64,209.88 v175.49,209.88 v174.47,209.88 v173.46,209.88 | R323.2 268.55,209.28 268.58,209.25 | R322.2 240.45,209.31 240.39,209.25 | R321.2 212.35,209.34 212.45,209.25 | R320.2 184.25,209.37 184.13,209.25 | R411.1 298.35,194.19 297.54,195 270.11,195 | 242.29,195 270.11,195 | 214.1,195 242.29,195 | 186.03,195 214.1,195 | R410.1 270.25,194.85 270.11,195 | R409.1 242.15,194.86 242.29,195 | R408.1 214.05,194.95 214.1,195 | R407.1 185.95,194.92 186.03,195 | R401.1 18.61,195 45.57,195 | 73.64,195 45.57,195 | 101.7,195 73.64,195 | 129.77,195 101.7,195 | 157.96,195 163.42,195 C401.1 166.59,193.84 v166.6,193.86 v167.62,193.86 v168.63,193.86 | 157.96,195 129.77,195 | 186.03,195 178.62,195 C402.1 175.5,193.84 v175.49,193.86 v174.47,193.86 v173.46,193.86 | R405.1 129.75,194.98 129.77,195 | R404.1 101.65,194.95 101.7,195 | R403.1 73.55,194.91 73.64,195
  Top 0.61: R402.1 45.45,194.88 45.57,195 | 15.64,147.38 R414.2 | 15.64,147.38 43.79,147.38 | 43.79,147.38 71.86,147.38 | 71.86,147.38 100.18,147.38 | 100.18,147.38 128.12,147.38 | 128.12,147.38 156.06,147.38 | 156.06,147.38 164.01,147.38 C405.1 164.52,147.88 v166.6,147.88 v167.62,147.88 v168.63,147.88 | R418.2 128.05,147.37 128.12,147.38 | R417.2 99.95,147.38 100.18,147.38 | R415.2 43.75,147.42 43.79,147.38 | R416.2 71.85,147.38 71.86,147.38 | 268.58,147.25 295.16,147.25 R424.2 | 240.39,147.25 268.58,147.25 | 212.45,147.25 240.39,147.25 | 184.13,147.25 212.45,147.25 | 184.13,147.25 178.28,147.25 C406.1 177.64,147.88 v175.49,147.88 v174.47,147.88 v173.46,147.88 | R423.2 268.55,147.28 268.58,147.25 | R422.2 240.45,147.31 240.39,147.25 | R421.2 212.35,147.34 212.45,147.25 | R420.2 184.25,147.37 184.13,147.25 | R511.1 298.35,132.19 298.35,133 | 270.11,133 298.35,133 | 242.29,133 270.11,133 | 214.1,133 242.29,133 | 186.03,133 214.1,133 | R510.1 270.25,132.85 270.11,133 | R509.1 242.15,132.86 242.29,133 | R508.1 214.05,132.95 214.1,133 | R507.1 185.95,132.92 186.03,133 | R501.1 18.61,133 45.57,133 | 73.64,133 45.57,133 | 101.7,133 73.64,133 | 129.77,133 101.7,133 | 157.84,133 163.42,133 C501.1 166.59,131.84 v166.6,131.86 v167.62,131.86 v168.63,131.86 | 157.84,133 129.77,133 | 186.03,133 178.62,133 C502.1 175.5,131.84 v175.49,131.86 v174.47,131.86 v173.46,131.86 | R505.1 129.75,132.98 129.77,133 | R504.1 101.65,132.95 101.7,133 | R503.1 73.55,132.91 73.64,133 | R502.1 45.45,132.88 45.57,133 | R514.2 17.02,85.38 43.79,85.38 | 71.86,85.38 43.79,85.38 | 100.18,85.38 71.86,85.38 | 128.12,85.38 100.18,85.38 | 156.19,85.38 164.01,85.38 C505.1 164.52,85.88 v166.6,85.88 v167.62,85.88 v168.63,85.88
  Top 0.61: 156.19,85.38 128.12,85.38 | R518.2 128.05,85.37 128.12,85.38 | R517.2 99.95,85.38 100.18,85.38 | R515.2 43.75,85.42 43.79,85.38 | R516.2 71.85,85.38 71.86,85.38 | 268.58,85.25 295.16,85.25 R524.2 | 240.39,85.25 268.58,85.25 | 212.45,85.25 240.39,85.25 | 184.13,85.25 212.45,85.25 | 184.13,85.25 178.28,85.25 C506.1 177.64,85.88 v175.49,85.88 v174.47,85.88 v173.46,85.88 | R523.2 268.55,85.28 268.58,85.25 | R522.2 240.45,85.31 240.39,85.25 | R521.2 212.35,85.34 212.45,85.25 | R520.2 184.25,85.37 184.13,85.25 | 15.64,147.38 9.18,147.38 7.6,145.8 7.6,83.44 9.63,81.41 9.63,69.34 8.61,68.33 J401A.3 J401A.1 J401.1 J401.3 | 298.35,133 308.71,133 310.13,131.57 310.13,84.48 306.3,80.64 J501.3 J501.1 J501A.1 J501A.3 | R106.1 157.85,380.89 157.96,381 | R119.2 156.15,333.41 156.19,333.38 | R206.1 157.84,317.74 157.84,319 | R219.2 156.19,272.74 156.19,271.38 | R319.2 156.15,209.47 156.06,209.38 | R306.1 157.85,256.99 157.84,257 | R406.1 157.96,193.74 157.96,195 | R419.2 156.15,147.47 156.06,147.38 | R506.1 157.85,132.99 157.84,133 | R519.2 156.15,85.41 156.19,85.38 | U601.7 278.48,62.22 278.36,62.1
  Top 1.27: v173.08,82.55 v174.09,82.55 v175.11,82.55 v176.12,82.55 v177.14,82.55 300.08,82.55 302.62,80.01 302.62,63.25 299.82,60.45 283.06,60.45 C604.1 C615.1 278.36,62.1
  Bottom 1.27: v166.6,379.86 v167.62,379.86 v168.63,379.86 171.68,379.86 | 171.68,379.86 v173.46,379.86 v174.47,379.86 v175.49,379.86 | v166.6,333.88 v167.62,333.88 v168.63,333.88 171.68,333.88 | 171.68,333.88 v173.46,333.88 v174.47,333.88 v175.49,333.88 | v166.6,317.86 v167.62,317.86 v168.63,317.86 171.68,317.86 | 171.68,317.86 v173.46,317.86 v174.47,317.86 v175.49,317.86 | v166.6,271.88 v167.62,271.88 v168.63,271.88 171.68,271.88 | 171.68,271.88 v173.46,271.88 v174.47,271.88 v175.49,271.88 | v166.6,255.86 v167.62,255.86 v168.63,255.86 171.68,255.86 | 171.68,255.86 v173.33,255.86 v174.35,255.86 v175.36,255.86 | v166.6,209.88 v167.62,209.88 v168.63,209.88 171.68,209.88 | 171.68,209.88 v173.46,209.88 v174.47,209.88 v175.49,209.88 | v166.6,193.86 v167.62,193.86 v168.63,193.86 171.68,193.86 | 171.68,193.86 v173.46,193.86 v174.47,193.86 v175.49,193.86 | v166.6,147.88 v167.62,147.88 v168.63,147.88 171.68,147.88 | 171.68,147.88 v173.46,147.88 v174.47,147.88 v175.49,147.88 | v166.6,131.86 v167.62,131.86 v168.63,131.86 171.68,131.86 | 171.68,131.86 v173.46,131.86 v174.47,131.86 v175.49,131.86 | v166.6,85.88 v167.62,85.88 v168.63,85.88 171.68,85.88 | 171.68,85.88 v173.46,85.88 v174.47,85.88 v175.49,85.88 | 171.68,333.88 171.68,351.79 175.49,355.6 175.49,358.78 171.68,362.59 171.68,379.86 | 171.68,317.86 171.68,333.88 | 171.68,271.88 171.68,317.86 | 171.68,255.86 171.68,271.88 | 171.68,209.88 171.68,227.33 175.49,231.14 175.49,234.95 171.68,238.76 171.68,255.86 | 171.68,193.86 171.68,209.88 | 171.68,147.88 171.68,193.86 | 171.68,147.88 171.68,131.86 | 171.68,131.86 171.68,115.57 175.49,111.76 175.49,106.68 171.68,102.87 171.68,85.88
  Bottom 1.27: 171.68,85.88 171.68,83.95 v173.08,82.55 v174.09,82.55 v175.11,82.55 v176.12,82.55 v177.14,82.55
VCC
  Top 0.61: J901.3 223.75,41.91 205.96,41.91 S901.2
  Bottom 0.406: C905.1 227.56,27.18 227.56,29.21 | 227.56,29.21 U901.34 U901.35 J901.3 | 227.56,29.21 C904.1
VCC+  (via drill 0.5)
  Top 0.61: v204.7,20.32 S901.1
  Bottom 0.61: v204.7,20.32 209.78,20.32 212.32,17.78 R901.1 R902.1

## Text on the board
Top: TOP | TOP | TOP | TOP
Bottom: BOT | BOT | BOT | BOT
tPlace: E | S | K | I | S | T | L | F | Ü | N | F | Z | E | H | N | Z | W | A | N | Z | I | G | D | R | E | I | V | I | E | R | T | E | L | T | G | N | A | C | H | V | O | R | J | M | H | A | L | B | Q | Z | W | Ö | L | F | P | Z | W | E | I | N | S | I | E | B | E | N | K | D | R | E | I | R | H | F | Ü | N | F | E | L | F | N | E | U | N | V | I | E | R | W | A | C | H | T | Z | E | H | N | R | S | B | S | E | C | H | S | F | M | U | H | R | tPL | DCF-77 Receiver | Minute | Bottom | Bottom | LEDs | Left | Right | Right | 3 | 4 | 3 | 4 | LCD + Keyboard | Minute | USB & Power | DCF-77 | LEDs | 1 | 2 | 1 | 2 | Top | Top | Rcv. | Left | tPL | tPL | Left | Right | LCD + Keyboard | PCB#201006002 | tPL
bPlace: DCF-77 | Rcv. | PA3 | PA4 | PA5 | PA6 | PE7 | PE6 | PA7 | PB0 | PE5 | PE4 | PE3 | PE2 | PB4 | PB5 | PE1 | PB6 | PE0 | PB7 | +3V3 | bPl | Minute | GND | LEDs | Right | Minute | LEDs | Left | bPl | bPl | bPl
